(* Logix 5000 AddOnInstructionDefinition export AMCI_5034_PTO_AM_Hold; software revision 37.00 *)

TYPE AMCI_5034_PTO_AM_Input_Data :
STRUCT
   ConnectionFaulted : DINT;
   MovingCW : BOOL;
   MovingCCW : BOOL;
   InHoldState : BOOL;
   Stopped : BOOL;
   AtHome : BOOL;
   Accelerating : BOOL;
   Decelerating : BOOL;
   MoveComplete : BOOL;
   HomeInvalid : BOOL;
   InvalidProfile : BOOL;
   PositionInvalid : BOOL;
   InputError : BOOL;
   CommandError : BOOL;
   ConfigurationError : BOOL;
   ModuleOK : BOOL;
   GeneralPurposeOutputStatus : BOOL;
   Input1Active : BOOL;
   Input2Active : BOOL;
   Input3Active : BOOL;
   Input4Active : BOOL;
   bit_20_reserved : BOOL;
   bit_21_reserved : BOOL;
   bit_22_reserved : BOOL;
   EncoderFollowerMode : BOOL;
   BlendMoveRunning : BOOL;
   BlendMoveAcknowledge : BOOL;
   MinimumRegistrationProgrammed : BOOL;
   EncoderMotionDirection : BOOL;
   MultipleInputsWithSameFunction : BOOL;
   FSCExceedsNumberOfDataBits : BOOL;
   AbsoluteEncoderSetupError : BOOL;
   bit_31_reserved : BOOL;
   CurrentPosition : DINT;
   EncoderPosition : DINT;
   CapturedPosition : DINT;
END_STRUCT
END_TYPE

TYPE AMCI_5034_PTO_AM_Output_Data :
STRUCT
   Command_Word : DINT;
   TargetPosition : DINT;
   TargetVelocity : UDINT;
   Acceleration : DINT;
   Deceleration : DINT;
END_STRUCT
END_TYPE

ADD_ON_INSTRUCTION AMCI_5034_PTO_AM_Hold   (* revision 1.0, vendor AMCI, ExecuteEnableInFalse *)
// AMCI Hold
// Revision note:
// 10/01/2025 Initial Release
// Help:
// AXIS INPUT DATA:  Input data from the AMCI 5034-PTO-AM.   Uses the AMCI_5034_PTO_Input_Data User Defined Data Type.
// AXIS OUTPUT DATA; Output data from the AOI to the AMCI 5034-PTO-AM.    Uses the AMCI_5034_PTO_Output_Data User Defined Data Type.
// EN (Enable) Set when rung is true, Reset when rung is false
// DN (Done) Set when command is sent to the motion device.  Reset when the rung is false.
// ER (Error) Set when a command or input error failed to clear.  Reset when the rung is false.
VAR_IN_OUT
   Axis_Input_Data : AMCI_5034_PTO_AM_Input_Data; {required}
   Axis_Output_Data : AMCI_5034_PTO_AM_Output_Data; {required}
END_VAR
VAR_OUTPUT
   EN : BOOL; {visible}   // set when rung with AOI is true
   DN : BOOL; {access Read Only, visible}   // set when reset error command sent to motion axis
   ER : BOOL; {access Read Only, visible}   // set when reset error command did not clear the error
END_VAR
VAR
   command_data_block : DINT[5];
        [0]   // Command Bits MSW
        [1]   // Command Bits LSW
        [2]   // Upper Target Position
        [3]   // Lower Target Position
        [4]   // Upper Programmed Speed
END_VAR

ROUTINE EnableInFalse   (* ladder *)
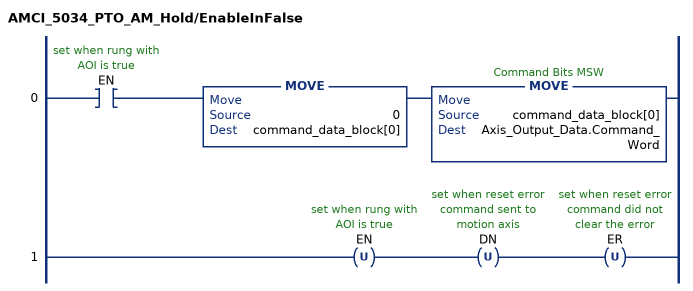
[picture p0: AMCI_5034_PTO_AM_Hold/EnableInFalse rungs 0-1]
   0: XIC(EN)MOVE(0,command_data_block[0])MOVE(command_data_block[0],Axis_Output_Data.Command_Word);
   1: OTU(EN)OTU(DN)OTU(ER);
END_ROUTINE

ROUTINE Logic   (* ladder *)
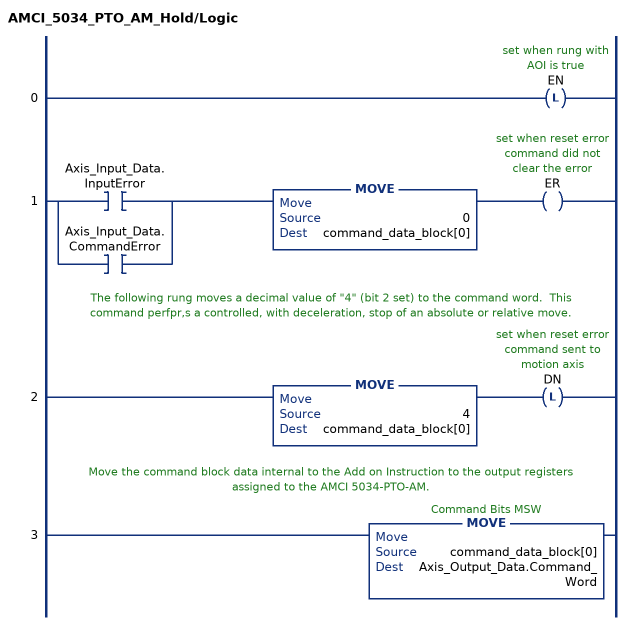
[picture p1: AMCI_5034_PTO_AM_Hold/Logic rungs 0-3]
   0: OTL(EN);
   1: [XIC(Axis_Input_Data.InputError) ,XIC(Axis_Input_Data.CommandError) ]MOVE(0,command_data_block[0])OTE(ER);
   // The following rung moves a decimal value of "4" (bit 2 set) to the command word.  This command perfpr,s a controlled, with deceleration, stop of an absolute or relative move.
   2: MOVE(4,command_data_block[0])OTL(DN);
   // Move the command block data internal to the Add on Instruction to the output registers assigned to the AMCI 5034-PTO-AM.
   3: MOVE(command_data_block[0],Axis_Output_Data.Command_Word);
END_ROUTINE
END_ADD_ON_INSTRUCTION
